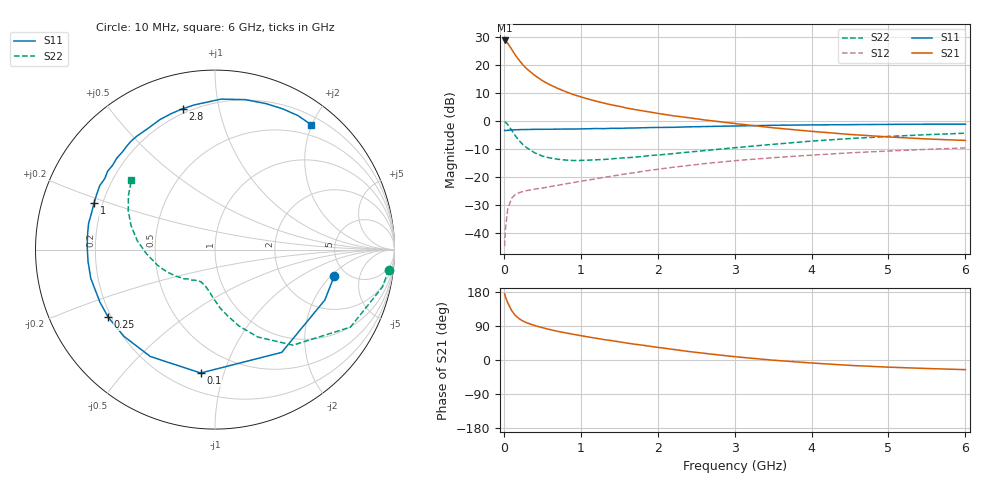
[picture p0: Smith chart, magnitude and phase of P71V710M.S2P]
! SIEMENS Small Signal Semiconductors
! BFP196
! Si NPN RF Bipolar Junction Transistor in SOT143
! VCE = 1.75 V  IC = 10 mA
! Common Emitter S-Parameters:  May  1996
# GHz  S  MA  R  50
!  f  S11  S21  S12  S22
! GHz  MAG  ANG  MAG  ANG  MAG  ANG  MAG  ANG
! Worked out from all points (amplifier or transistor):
!   36 points, 10 MHz to 6 GHz, reference 50 ohm
!   highest |S21| = 28.9 dB at 10 MHz (marker M1)
!   |S21| within 3 dB of that: start of sweep to 98.02 MHz
!   unconditionally stable (mu >= 1): 860.2 MHz to 3.38 GHz
!   at 250 MHz: K = 0.40, MSG = 22.7 dB, |S12| = -25.2 dB
!   at 1.4 GHz: K = 1.14, MAG = 10.5 dB, |S12| = -19.8 dB
!   at 6 GHz: K = 0.99, MSG = 1.3 dB, |S12| = -9.6 dB
!   S11 on the Smith chart (normalised r, x): 10 MHz: 3.96, -2.20; 100 MHz: 0.32, -0.84; 250 MHz: 0.19, -0.28; 1 GHz: 0.17, +0.18; 2.8 GHz: 0.17, +0.78; 6 GHz: 0.33, +1.99
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0.01  0.6799 -12.7  27.87 174.7  0.0057 84.1  0.9741 -6.6
0.02  0.6735 -24.6  27.22 167.4  0.0114 76.9  0.956 -12.6
0.05  0.6827 -57.0  24.86 151.2  0.0261 65.4  0.8693 -29.8
0.1  0.6921 -96.6  19.55 130.9  0.0411 49.2  0.6871 -50.8
0.15  0.6962 -121.2  15.21 117.4  0.0481 39.8  0.5415 -64.0
0.2  0.7007 -136.4  12.29 108.9  0.0519 35.2  0.444 -72.8
0.25  0.7041 -147.6  10.1 102.6  0.0548 32.7  0.3753 -79.2
0.3  0.7048 -155.4  8.604 98.0  0.0566 31.8  0.3309 -84.5
0.4  0.7105 -167.0  6.615 91.0  0.0601 31.8  0.2697 -92.2
0.5  0.7104 -174.7  5.309 85.4  0.0627 33.1  0.2357 -97.9
0.6  0.7125 178.4  4.464 80.3  0.0666 34.4  0.2175 -102.5
0.7  0.7155 172.6  3.856 75.6  0.0704 36.2  0.2064 -106.5
0.8  0.7192 168.2  3.379 71.8  0.0744 37.5  0.2 -110.5
1  0.7223 158.8  2.713 64.3  0.083 40.1  0.1965 -115.9
1.1  0.7276 154.9  2.475 60.7  0.0875 41.1  0.199 -118.5
1.6  0.7474 137.1  1.708 44.7  0.1136 43.3  0.2203 -131.1
2.2  0.7715 119.0  1.244 28.0  0.1483 41.4  0.2606 -145.0
2.8  0.8056 102.8  0.975 13.2  0.1828 36.7  0.3128 -160.1
3.5  0.839 87.7  0.757 -0.5  0.2202 29.2  0.3823 -176.5
4.5  0.8614 70.8  0.575 -14.2  0.2689 18.3  0.4855 164.2
5.5  0.8782 58.2  0.477 -22.4  0.3108 7.0  0.5695 147.8
6  0.8779 52.4  0.449 -25.5  0.3296 0.9  0.6051 140.4
